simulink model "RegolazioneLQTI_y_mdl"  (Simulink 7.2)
settings: Solver=ode45  StartTime=0.0  StopTime=10.0  RelTol=1e-3
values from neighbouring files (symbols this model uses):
  A = [0 1; -2 1]    [RegolazioneOttimaTempoInfinita_Integrale.m]    (also in RegolazioneOttimaTempoInfinita_TempoDiscreto.m; RegolazioneOttimaTempoInfinita_uscita.m; RegolazioneOttimaTempoInfinita_uscita_osservatore.m; RegolazioneOttimaTempoInfinita.m)
  B = [0; 1]    [RegolazioneOttimaTempoInfinita_Integrale.m]    (also in RegolazioneOttimaTempoInfinita_TempoDiscreto.m; RegolazioneOttimaTempoInfinita_uscita.m; RegolazioneOttimaTempoInfinita_uscita_osservatore.m; RegolazioneOttimaTempoInfinita.m)
  C = [1 0]    [RegolazioneOttimaTempoInfinita_Integrale.m]    (also in RegolazioneOttimaTempoInfinita_TempoDiscreto.m; RegolazioneOttimaTempoInfinita_uscita.m = [0 1]; RegolazioneOttimaTempoInfinita_uscita_osservatore.m = [0 1]; RegolazioneOttimaTempoInfinita.m)
  X0 = [2;-3]    [RegolazioneOttimaTempoInfinita_Integrale.m]    (also in RegolazioneOttimaTempoInfinita_TempoDiscreto.m; RegolazioneOttimaTempoInfinita_uscita.m; RegolazioneOttimaTempoInfinita_uscita_osservatore.m; RegolazioneOttimaTempoInfinita.m)
undefined symbols (not defined in the file or in its folder): K

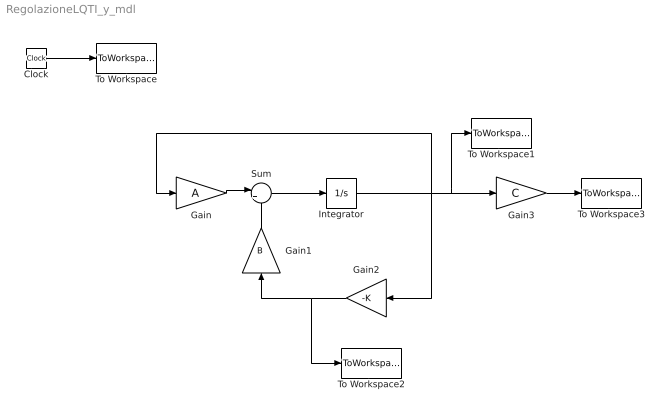
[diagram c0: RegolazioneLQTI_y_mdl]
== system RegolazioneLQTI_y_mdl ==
  Clock : Clock
  Gain : Gain  Gain=A  Multiplication=Matrix(K*u)  ParameterDataType=sfix(16)  ParameterScaling=2^0  OutDataType=sfix(16)  OutScaling=2^0
  Gain1 : Gain  Orientation=up  Gain=B  Multiplication=Matrix(K*u)  ParameterDataType=sfix(16)  ParameterScaling=2^0  OutDataType=sfix(16)  OutScaling=2^0
  Gain2 : Gain  Orientation=left  Gain=-K  Multiplication=Matrix(K*u)  ParameterDataType=sfix(16)  ParameterScaling=2^0  OutDataType=sfix(16)  OutScaling=2^0
  Gain3 : Gain  Gain=C  Multiplication=Matrix(K*u)  ParameterDataType=sfix(16)  ParameterScaling=2^0  OutDataType=sfix(16)  OutScaling=2^0
  Integrator : Integrator  InitialCondition=X0
  Sum : Sum  Inputs=|++  OutDataType=sfix(16)  OutScaling=2^0
  To Workspace : ToWorkspace  VariableName=time  SampleTime=-1  SaveFormat=Array
  To Workspace1 : ToWorkspace  VariableName=X  SampleTime=-1  SaveFormat=Array
  To Workspace2 : ToWorkspace  VariableName=u  SampleTime=-1  SaveFormat=Array
  To Workspace3 : ToWorkspace  VariableName=y  SampleTime=-1  SaveFormat=Array
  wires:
  Gain/1 -> Sum/1
  Integrator/1 -> Gain/1, Gain2/1, To Workspace1/1, Gain3/1
  Gain1/1 -> Sum/2
  Gain2/1 -> Gain1/1, To Workspace2/1
  Sum/1 -> Integrator/1
  Clock/1 -> To Workspace/1
  Gain3/1 -> To Workspace3/1
